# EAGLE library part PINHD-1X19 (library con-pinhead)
PIN HEADER
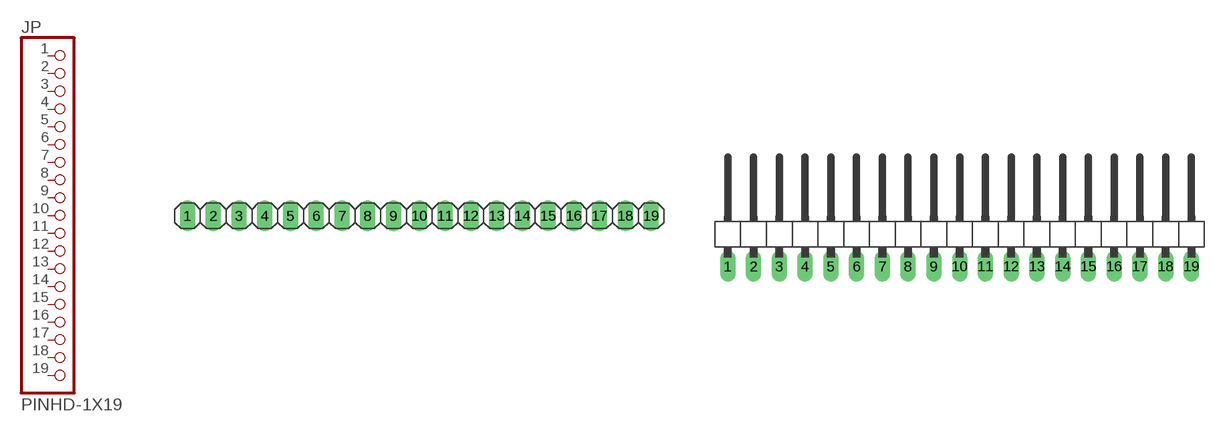
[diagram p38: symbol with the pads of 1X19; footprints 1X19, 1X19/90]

Designator prefix JP

## PINHD-1X19_2.54  [1X19]
1  1  pas
2  2  pas
3  3  pas
4  4  pas
5  5  pas
6  6  pas
7  7  pas
8  8  pas
9  9  pas
10  10  pas
11  11  pas
12  12  pas
13  13  pas
14  14  pas
15  15  pas
16  16  pas
17  17  pas
18  18  pas
19  19  pas

## PINHD-1X19_2.54-90°  [1X19/90]
Pads as for 1X19

## PINHD-1X19_2.00  [1X19M]
Pads as for 1X19

## PINHD-1X19_2.54-SMD  [1X19SMD]
Pads as for 1X19

## PINHD-1X19  [1X19SMD/90]
Pads as for 1X19

## Footprint 1X19 (pad centres in mm)
PIN HEADER - 2.54
drill 1.016 long: 1 -22.86,0; 2 -20.32,0; 3 -17.78,0; 4 -15.24,0; 5 -12.7,0; 6 -10.16,0; 7 -7.62,0; 8 -5.08,0; 9 -2.54,0; 10 0,0; 11 2.54,0; 12 5.08,0; 13 7.62,0; 14 10.16,0; 15 12.7,0; 16 15.24,0; 17 17.78,0; 18 20.32,0; 19 22.86,0

## Footprint 1X19/90 (pad centres in mm)
PIN HEADER - 2.54 90°
drill 1.016 long: 1 -22.86,-3.81; 2 -20.32,-3.81; 3 -17.78,-3.81; 4 -15.24,-3.81; 5 -12.7,-3.81; 6 -10.16,-3.81; 7 -7.62,-3.81; 8 -5.08,-3.81; 9 -2.54,-3.81; 10 0,-3.81; 11 2.54,-3.81; 12 5.08,-3.81; 13 7.62,-3.81; 14 10.16,-3.81; 15 12.7,-3.81; 16 15.24,-3.81; 17 17.78,-3.81; 18 20.32,-3.81; 19 22.86,-3.81

## Footprint 1X19M (pad centres in mm)
PIN HEADER - 2
drill 0.914 square: 1 -18,0
drill 0.914: 2 -16,0; 3 -14,0; 4 -12,0; 5 -10,0; 6 -8,0; 7 -6,0; 8 -4,0; 9 -2,0; 10 0,0; 11 2,0; 12 4,0; 13 6,0; 14 8,0; 15 10,0; 16 12,0; 17 14,0; 18 16,0; 19 18,0

## Footprint 1X19SMD (pad centres in mm)
PIN HEADER - 2.54 SMD
smd 1.016 x 3.302: 1 -1.27,1.27; 2 1.27,-1.27; 3 3.81,1.27; 4 6.35,-1.27; 5 8.89,1.27; 6 11.43,-1.27; 7 13.97,1.27; 8 16.51,-1.27; 9 19.05,1.27; 10 21.59,-1.27; 11 24.13,1.27; 12 26.67,-1.27; 13 29.21,1.27; 14 31.75,-1.27; 15 34.29,1.27; 16 36.83,-1.27; 17 39.37,1.27; 18 41.91,-1.27; 19 44.45,1.27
